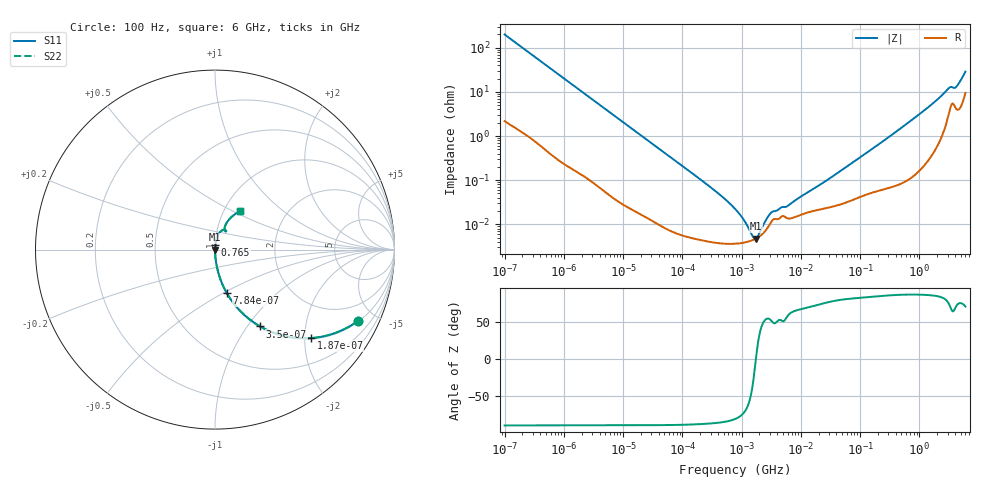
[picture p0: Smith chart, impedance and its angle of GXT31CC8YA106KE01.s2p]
!Murata Part Number: GXT31CC8YA106KE01
!These Parameters are Measured in Series Mode Connection
!Data Generated on Jan 08, 2026
!  o--ll--o
!Port1  Port2
!  o------o
!Operation Temp=25[degC], DC Bias Voltage=0[V]
!Freq. Start=100[Hz] Stop=6[GHz] 401[Steps]
# Hz S RI R 50
!Freq.(Hz) S11(Real) S11(Imag) S21(Real) S21(Imag) S12(Real) S12(Imag) S22(Real) S22(Imag)
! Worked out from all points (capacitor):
!   401 points, 100 Hz to 6 GHz, reference 50 ohm
!   read as one part in series: C = 7.93 uF near 109 Hz
!   lowest |Z| = 4.73 mohm at 1.734 MHz (marker M1)
!   series resonance near 1.744 MHz, so ESL is about 1 nH
!   S11 on the Smith chart (normalised r, x): 100 Hz: 1.04, -4.00; 187 Hz: 1.03, -2.15; 350 Hz: 1.01, -1.15; 784 Hz: 1.01, -0.52; 765 MHz: 1.00, +0.05; 6 GHz: 1.19, +0.54
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100  0.7976 -0.3964  0.2024 0.3964  0.2024 0.3964  0.7976 -0.3964
187  0.5351 -0.4929  0.4649 0.4929  0.4649 0.4929  0.5351 -0.4929
350  0.2523 -0.4283  0.7477 0.4283  0.7477 0.4283  0.2523 -0.4283
524  0.133 -0.3338  0.867 0.3338  0.867 0.3338  0.133 -0.3338
784  0.0653 -0.2415  0.9347 0.2415  0.9347 0.2415  0.0653 -0.2415
2008  0.0115 -0.1006  0.9885 0.1006  0.9885 0.1006  0.0115 -0.1006
6433  0.00144 -0.0321  0.9986 0.0321  0.9986 0.0321  0.00144 -0.0321
40335  0.000124 -0.0052  0.9999 0.0052  0.9999 0.0052  0.000124 -0.0052
330837  3.92e-05 -0.000621  1 0.000621  1 0.000621  3.92e-05 -0.000621
774597  3.63e-05 -0.000222  1 0.000222  1 0.000222  3.63e-05 -0.000222
1212075  3.96e-05 -9.18e-05  1 9.18e-05  1 9.18e-05  3.96e-05 -9.18e-05
1734173  4.73e-05 -1.4e-06  1 1.4e-06  1 1.4e-06  4.73e-05 -1.4e-06
2268635  6.09e-05 6.68e-05  0.9999 -6.68e-05  0.9999 -6.68e-05  6.09e-05 6.68e-05
3245845  0.000119 0.000147  0.9999 -0.000147  0.9999 -0.000147  0.000119 0.000147
6075234  0.000136 0.000226  0.9999 -0.000226  0.9999 -0.000226  0.000136 0.000226
1.555665e7  0.000198 0.000578  0.9998 -0.000578  0.9998 -0.000578  0.000198 0.000578
3.124326e8  0.000763 0.00966  0.9992 -0.00966  0.9992 -0.00966  0.000763 0.00966
7.650043e8  0.00174 0.0236  0.9983 -0.0236  0.9983 -0.0236  0.00174 0.0236
1.712697e9  0.00706 0.0548  0.9929 -0.0548  0.9929 -0.0548  0.00706 0.0548
3.065283e9  0.0386 0.1065  0.9614 -0.1065  0.9614 -0.1065  0.0386 0.1065
4.193612e9  0.0531 0.1119  0.9469 -0.1119  0.9469 -0.1119  0.0531 0.1119
6e9  0.1393 0.214  0.8607 -0.214  0.8607 -0.214  0.1393 0.214
